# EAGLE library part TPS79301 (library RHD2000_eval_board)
Texas Instruments TPS79301 adjustable regulator
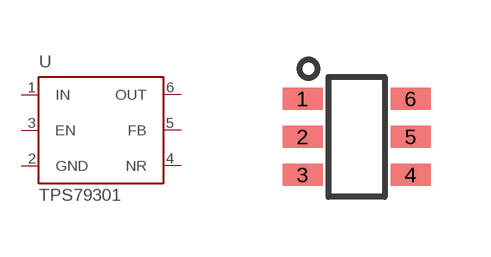
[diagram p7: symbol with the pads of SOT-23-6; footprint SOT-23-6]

Designator prefix U

## TPS79301  [SOT-23-6]
1  IN  pwr
2  GND  pwr
3  EN  in
4  NR  pas
5  FB  in
6  OUT  pwr

## Footprint SOT-23-6 (pad centres in mm)
smd 1 x 0.55: 1 -1.35,0.95; 2 -1.35,0; 3 -1.35,-0.95; 4 1.35,-0.95; 5 1.35,0; 6 1.35,0.95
